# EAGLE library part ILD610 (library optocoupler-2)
SIEMENS OPTO COUPLER
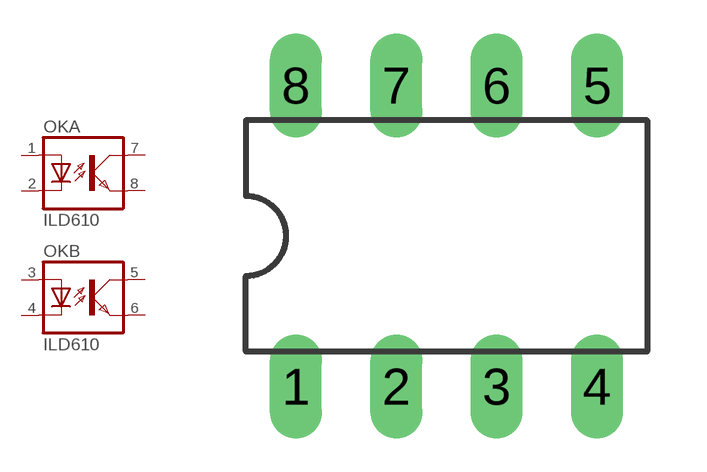
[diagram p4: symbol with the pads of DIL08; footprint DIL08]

Designator prefix OK; gates A=OK B=OK

## ILD610  [DIL08]
1  A:A  pas
2  A:C  pas
3  B:A  pas
4  B:C  pas
5  B:COL  pas
6  B:EMIT  pas
7  A:COL  pas
8  A:EMIT  pas

## Footprint DIL08 (pad centres in mm)
Dual In Line Package
drill 0.813 long: 1 -3.81,-3.81; 2 -1.27,-3.81; 3 1.27,-3.81; 4 3.81,-3.81; 5 3.81,3.81; 6 1.27,3.81; 7 -1.27,3.81; 8 -3.81,3.81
